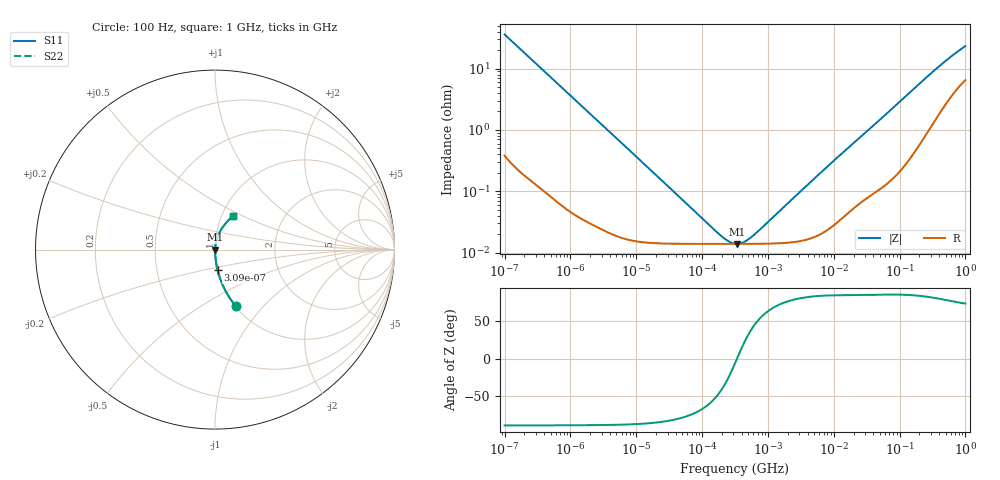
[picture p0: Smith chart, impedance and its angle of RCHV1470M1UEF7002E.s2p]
! RCHV1470M1UEF7002E  S-PARAMETER MODEL  (AEC-Q200 qualified)
! Model Generated by ELNA Corporation (http://www.ty-top.com)
! Version 1.0
! ELNA Control No. 240229
! Copyright (c) 2024 ELNA CO.,LTD. All Rights Reserved.
! Products Name : CONDUCTIVE POLYMER HYBRID ALUMINUM ELECTROLYTIC CAPACITORS
! Characteristics :
!  Capacitance  :  47uF  ,  Rated voltage  :  50V
!  Operating Temp. Range  :  -55 to +105 degC  ,  Endurance  :  10000hr at 105 degC
!  Dimension D  :  8mm  ,  Dimension L  :  8.7mm
! Frequency Range : 100Hz - 1GHz
! External Node Assignments :
!  1  o---| |---o  2
# MHz S RI R 50
!Freq[MHz].  S11 Real  S11 Imag  S21 Real  S21 Imag  S12 Real  S12 Imag  S22 Real  S22 Imag
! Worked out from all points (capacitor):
!   401 points, 100 Hz to 1 GHz, reference 50 ohm
!   read as one part in series: C = 44.3 uF near 108 Hz
!   lowest |Z| = 13.9 mohm at 342.8 kHz (marker M1)
!   series resonance near 339.2 kHz, so ESL is about 5 nH
!   S11 on the Smith chart (normalised r, x): 100 Hz: 1.01, -0.72; 309 Hz: 1.00, -0.23; 1 GHz: 1.13, +0.45
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0.0001  0.1168 -0.3159  0.8832 0.3159  0.8832 0.3159  0.1168 -0.3159
0.000113  0.0944 -0.2872  0.9056 0.2872  0.9056 0.2872  0.0944 -0.2872
0.000162  0.0487 -0.2104  0.9513 0.2104  0.9513 0.2104  0.0487 -0.2104
0.000309  0.0146 -0.1148  0.9854 0.1148  0.9854 0.1148  0.0146 -0.1148
0.000613  0.00415 -0.0588  0.9958 0.0588  0.9958 0.0588  0.00415 -0.0588
0.001488  0.00095 -0.0244  0.999 0.0244  0.999 0.0244  0.00095 -0.0244
0.004241  0.000275 -0.00863  0.9997 0.00863  0.9997 0.00863  0.000275 -0.00863
0.022131  0.000145 -0.00165  0.9999 0.00165  0.9999 0.00165  0.000145 -0.00165
0.179887  0.000139 -0.000147  0.9999 0.000147  0.9999 0.000147  0.000139 -0.000147
0.248313  0.000139 -6.87e-05  0.9999 6.87e-05  0.9999 6.87e-05  0.000139 -6.87e-05
0.316228  0.000139 -1.52e-05  0.9999 1.52e-05  0.9999 1.52e-05  0.000139 -1.52e-05
0.342768  0.000139 2.31e-06  0.9999 -2.31e-06  0.9999 -2.31e-06  0.000139 2.31e-06
0.386812  0.000139 2.86e-05  0.9999 -2.86e-05  0.9999 -2.86e-05  0.000139 2.86e-05
0.436516  0.000139 5.53e-05  0.9999 -5.53e-05  0.9999 -5.53e-05  0.000139 5.53e-05
0.60256  0.00014 0.000132  0.9999 -0.000132  0.9999 -0.000132  0.00014 0.000132
4.704354  0.000177 0.00149  0.9998 -0.00149  0.9998 -0.00149  0.000177 0.00149
11.88502  0.000339 0.0037  0.9997 -0.0037  0.9997 -0.0037  0.000339 0.0037
69.9842  0.00183 0.0201  0.9982 -0.0201  0.9982 -0.0201  0.00183 0.0201
176.8072  0.0071 0.0494  0.9929 -0.0494  0.9929 -0.0494  0.0071 0.0494
380.1894  0.0264 0.0985  0.9736 -0.0985  0.9736 -0.0985  0.0264 0.0985
668.3439  0.0622 0.1493  0.9378 -0.1493  0.9378 -0.1493  0.0622 0.1493
1000  0.1004 0.1889  0.8996 -0.1889  0.8996 -0.1889  0.1004 0.1889
